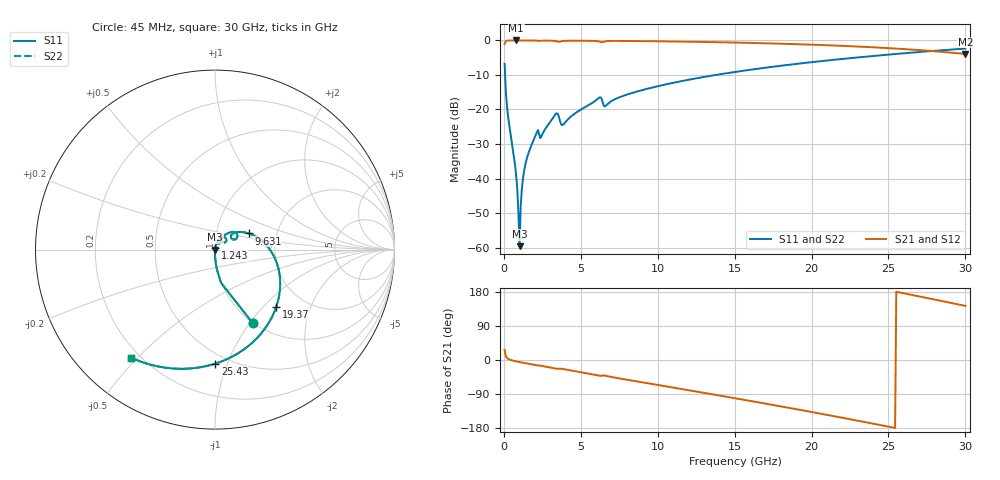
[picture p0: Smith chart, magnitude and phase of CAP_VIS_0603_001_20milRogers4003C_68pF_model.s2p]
! S-parameter model data by Modelithics Inc.  support@modelithics.com  813-866-6335  Tampa FL USA
! S-Parameter data specifications:
! Substrate: 20-mil Rogers 4003C, substrate thickness, H=0.508mm, Dielectric constant, Er=3.75
! PCB Mounting Pad Footprint: Pad width, PadW=0.90mm , Pad length, PadL=1.00mm , Pad gap, PadG (edge-to-edge)=1.00mm , Reference planes=3.0mm apart
! Created Wed Nov 18 13:29:59 2015
# hz S ma R 50
! 2 Port Network Data from SP1.SP block
! freq  magS11  angS11  magS21  angS21  magS12  angS12  magS22  angS22
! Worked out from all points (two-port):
!   401 points, 45 MHz to 30 GHz, reference 50 ohm
!   highest |S21| = -0.01 dB at 793.9 MHz (marker M1); lowest = -3.9 dB at 30 GHz (marker M2)
!   |S21| within 3 dB of the highest: start of sweep to 27.63 GHz
!   lowest |S11| = -59.6 dB at 1.019 GHz (marker M3), VSWR 1.00, Z = 50.1 + j0.0495 ohm
!   |S11| at or under -10 dB: 76.36 MHz to 13.78 GHz (13.7 GHz wide, 198 % of centre)
!   |S22| runs from -59.6 to -2.4 dB; largest |S21 - S12| = 0
!   S11 on the Smith chart (normalised r, x): 45 MHz: 1.00, -1.03; 1.243 GHz: 1.00, +0.02; 9.631 GHz: 1.43, +0.27; 19.37 GHz: 1.46, -1.19; 25.43 GHz: 0.43, -0.91; 30 GHz: 0.17, -0.48
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4.5e7  0.4594 -62.9  0.888 27.1  0.888 27.1  0.4594 -62.9
3.4455e8  0.05972 -87.9  0.9977 1.6  0.9977 1.6  0.05972 -87.9
7.93875e8  0.0112 -89.7  0.9991 -3.6  0.9991 -3.6  0.0112 -89.7
8.687625e8  0.006943 -87.6  0.9991 -4.2  0.9991 -4.2  0.006943 -87.6
1.018538e9  0.001047 28.2  0.999 -5.5  0.999 -5.5  0.001047 28.2
1.168312e9  0.007163 75.8  0.9989 -6.6  0.9989 -6.6  0.007163 75.8
1.2432e9  0.01017 77.3  0.9989 -7.2  0.9989 -7.2  0.01017 77.3
1.54275e9  0.02136 77.4  0.9985 -9.5  0.9985 -9.5  0.02136 77.4
2.066962e9  0.04232 72.0  0.9956 -13.5  0.9956 -13.5  0.04232 72.0
2.516288e9  0.04481 68.5  0.9945 -16.0  0.9945 -16.0  0.04481 68.5
3.34005e9  0.08443 56.1  0.9798 -22.6  0.9798 -22.6  0.08443 56.1
3.864262e9  0.06052 50.7  0.982 -24.0  0.982 -24.0  0.06052 50.7
5.062462e9  0.1014 54.9  0.9903 -32.8  0.9903 -32.8  0.1014 54.9
6.185775e9  0.1478 40.7  0.9684 -41.4  0.9684 -41.4  0.1478 40.7
9.6306e9  0.2076 25.8  0.9739 -63.3  0.9739 -63.3  0.2076 25.8
1.007992e10  0.2192 22.7  0.9713 -66.4  0.9713 -66.4  0.2192 22.7
1.50225e10  0.3494 -11.5  0.9317 -100.9  0.9317 -100.9  0.3494 -11.5
1.936598e10  0.4668 -43.0  0.8779 -132.4  0.8779 -132.4  0.4668 -43.0
2.003996e10  0.4853 -48.0  0.8677 -137.5  0.8677 -137.5  0.4853 -48.0
2.505742e10  0.6248 -86.9  0.7724 -176.4  0.7724 -176.4  0.6248 -86.9
2.543186e10  0.6354 -89.9  0.7637 -179.4  0.7637 -179.4  0.6354 -89.9
3e10  0.7618 -127.7  0.6369 142.8  0.6369 142.8  0.7618 -127.7
